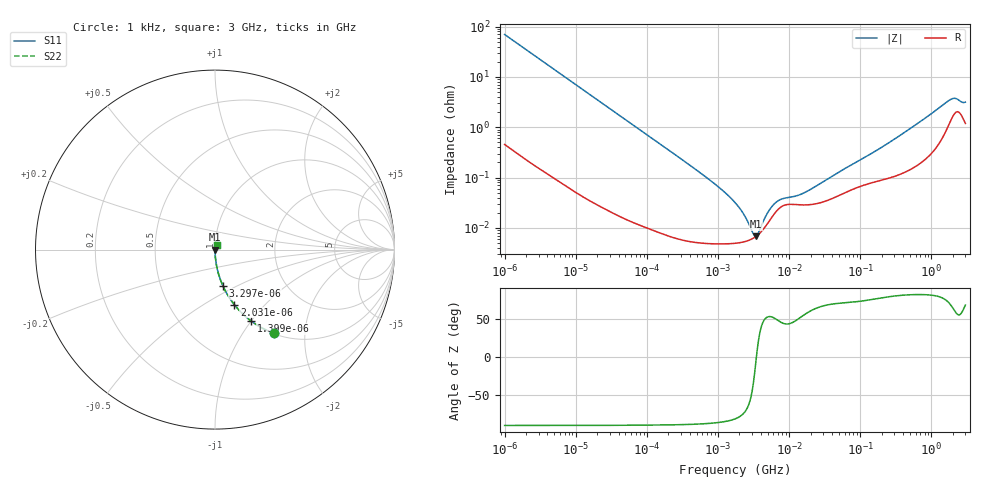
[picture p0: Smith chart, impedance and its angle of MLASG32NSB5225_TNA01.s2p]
! MLASG32NSB5225_TNA01  S-PARAMETER MODEL  ( Standard Model )
! Model Generated by TAIYO YUDEN Corporation (http://www.ty-top.com)
! Version 1.0
! TAIYO YUDEN Control No. 220601
! Copyright(c) 2008 TAIYO YUDEN CO.,LTD. All Rights Reserved.
! Product Description (link to TY-COMPAS)
! https://ds.yuden.co.jp/TYCOMPAS/or/detail?pn=MLASG32NSB5225KTNA01&u=M
! Products Name : Multilayer Ceramic Capacitors
! Characteristics :
!  Capacitance : 2.2 [uF] , Rated Voltage : 35 [V] , TCC : B / X5R
!  Case Size : 3.2 x 2.5 / 0.126 x 0.098 [mm/inch] , Thickness : 1.9 / 0.075 [mm/inch]
!  (Conditions: Temperature = 25 [degC] , DC Bias Voltage = 0 [V])
! External Node Assignments :
!  1  o---| |---o  2
! GND o---------o GND
! Frequency Range : 1kHz  -  3GHz  [ 401 STEP ]
# MHZ S RI R 50
! Freq[MHz].  S11 Real  S11 Imag  S21 Real  S21 Imag  S12 Real  S12 Imag  S22 Real  S22 Imag
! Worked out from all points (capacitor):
!   401 points, 1 kHz to 3 GHz, reference 50 ohm
!   read as one part in series: C = 2.28 uF near 1.077 kHz
!   lowest |Z| = 6.78 mohm at 3.389 MHz (marker M1)
!   series resonance near 3.464 MHz, so ESL is about 920 pH
!   S11 on the Smith chart (normalised r, x): 1 kHz: 1.01, -1.39; 1.399 kHz: 1.01, -1.00; 2.031 kHz: 1.00, -0.69; 3.297 kHz: 1.00, -0.42; 3 GHz: 1.02, +0.06
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0.001  0.3273 -0.466  0.6727 0.466  0.6727 0.466  0.3273 -0.466
0.001399  0.2004 -0.3971  0.7996 0.3971  0.7996 0.3971  0.2004 -0.3971
0.002031  0.1072 -0.3061  0.8928 0.3061  0.8928 0.3061  0.1072 -0.3061
0.003297  0.0443 -0.2024  0.9557 0.2024  0.9557 0.2024  0.0443 -0.2024
0.005988  0.0143 -0.1153  0.9857 0.1153  0.9857 0.1153  0.0143 -0.1153
0.01216  0.00375 -0.0576  0.9962 0.0576  0.9962 0.0576  0.00375 -0.0576
0.147855  0.000104 -0.0048  0.9999 0.0048  0.9999 0.0048  0.000104 -0.0048
0.791611  4.92e-05 -0.00086  1 0.00086  1 0.00086  4.92e-05 -0.00086
1.732051  4.95e-05 -0.000315  1 0.000315  1 0.000315  4.95e-05 -0.000315
2.166294  5.17e-05 -0.000207  0.9999 0.000207  0.9999 0.000207  5.17e-05 -0.000207
2.812335  5.78e-05 -9.03e-05  0.9999 9.03e-05  0.9999 9.03e-05  5.78e-05 -9.03e-05
3.03007  6.08e-05 -5.8e-05  0.9999 5.8e-05  0.9999 5.8e-05  6.08e-05 -5.8e-05
3.388684  6.71e-05 -9.54e-06  0.9999 9.54e-06  0.9999 9.54e-06  6.71e-05 -9.54e-06
3.93371  8.06e-05 5.57e-05  0.9999 -5.57e-05  0.9999 -5.57e-05  8.06e-05 5.57e-05
5.30084  0.000139 0.000183  0.9999 -0.000183  0.9999 -0.000183  0.000139 0.000183
6.881678  0.000228 0.000253  0.9998 -0.000253  0.9998 -0.000253  0.000228 0.000253
13.97519  0.000287 0.000351  0.9997 -0.000351  0.9997 -0.000351  0.000287 0.000351
21.06097  0.000293 0.000532  0.9997 -0.000532  0.9997 -0.000532  0.000293 0.000532
256.0921  0.001 0.00488  0.999 -0.00488  0.999 -0.00488  0.001 0.00488
1847.629  0.0139 0.0321  0.9861 -0.0321  0.9861 -0.0321  0.0139 0.0321
2144.796  0.0197 0.031  0.9803 -0.031  0.9803 -0.031  0.0197 0.031
3000  0.0126 0.0284  0.9874 -0.0284  0.9874 -0.0284  0.0126 0.0284
